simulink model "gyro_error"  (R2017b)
settings: Solver=VariableStepAuto  StartTime=0.0  StopTime=10.0  RelTol=1e-3
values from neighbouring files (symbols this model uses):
  Kg = 15/pi    (= 4.77464829276)    [init.m]
  lg = 0.7    [init.m]
  wg = 200*pi    (= 628.318530718)    [init.m]
undefined symbols (not defined in the file or in its folder): wg2

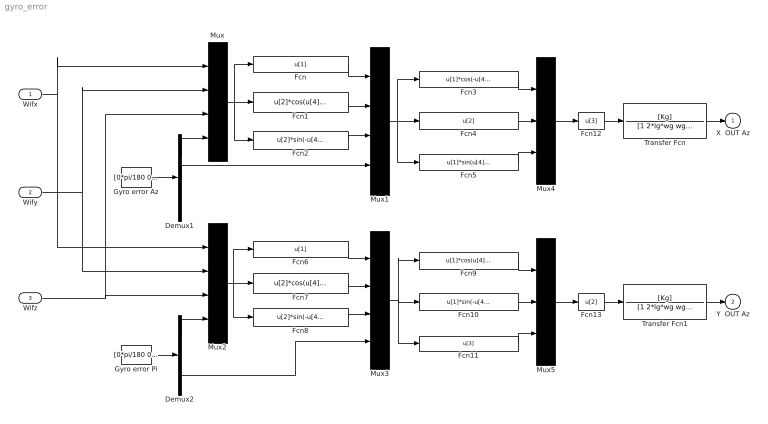
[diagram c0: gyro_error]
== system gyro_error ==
  Wifx : Inport
  Wify : Inport  Port=2
  Wifz : Inport  Port=3
  Demux1 : Demux  Outputs=3
  Demux2 : Demux  Outputs=3
  Fcn : Fcn  Expr=u[1]
  Fcn1 : Fcn  Expr=u[2]*cos(u[4])+u[3]*sin(u[4])
  Fcn10 : Fcn  Expr=u[1]*sin(-u[4])+u[2]*cos(u[4])
  Fcn11 : Fcn  Expr=u[3]
  Fcn12 : Fcn  Expr=u[3]
  Fcn13 : Fcn  Expr=u[2]
  Fcn2 : Fcn  Expr=u[2]*sin(-u[4])+u[3]*cos(u[4])
  Fcn3 : Fcn  Expr=u[1]*cos(-u[4])+u[3]*sin(-u[4])
  Fcn4 : Fcn  Expr=u[2]
  Fcn5 : Fcn  Expr=u[1]*sin(u[4])+u[3]*cos(u[4])
  Fcn6 : Fcn  Expr=u[1]
  Fcn7 : Fcn  Expr=u[2]*cos(u[4])+u[3]*sin(u[4])
  Fcn8 : Fcn  Expr=u[2]*sin(-u[4])+u[3]*cos(u[4])
  Fcn9 : Fcn  Expr=u[1]*cos(u[4])+u[2]*sin(u[4])
  Gyro error Az : Constant  Value=[0*pi/180 0*pi/180 0*pi/180]'
  Gyro error Pi : Constant  Value=[0*pi/180 0*pi/180 0*pi/180]'
  Mux{,1..3} (4 alike) : Mux
  Mux4 : Mux  Inputs=3
  Mux5 : Mux  Inputs=3
  Transfer Fcn : TransferFcn  Numerator=[Kg]  Denominator=[1 2*lg*wg wg2]
  Transfer Fcn1 : TransferFcn  Numerator=[Kg]  Denominator=[1 2*lg*wg wg2]
  X  OUT Az : Outport
  Y  OUT Az : Outport  Port=2
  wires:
  Gyro error Az/1 -> Demux1/1
  Gyro error Pi/1 -> Demux2/1
  Mux/1 -> Fcn/1, Fcn1/1, Fcn2/1
  Wifx/1 -> Mux/1, Mux2/1
  Wify/1 -> Mux/2, Mux2/2
  Wifz/1 -> Mux/3, Mux2/3
  Demux1/1 -> Mux/4
  Mux1/1 -> Fcn3/1, Fcn4/1, Fcn5/1
  Fcn/1 -> Mux1/1
  Fcn1/1 -> Mux1/2
  Fcn2/1 -> Mux1/3
  Demux1/2 -> Mux1/4
  Mux3/1 -> Fcn9/1, Fcn10/1, Fcn11/1
  Demux2/1 -> Mux2/4
  Fcn6/1 -> Mux3/1
  Mux2/1 -> Fcn8/1, Fcn7/1, Fcn6/1
  Fcn7/1 -> Mux3/2
  Fcn8/1 -> Mux3/3
  Demux2/3 -> Mux3/4
  Fcn3/1 -> Mux4/1
  Fcn4/1 -> Mux4/2
  Fcn5/1 -> Mux4/3
  Fcn9/1 -> Mux5/1
  Fcn10/1 -> Mux5/2
  Fcn11/1 -> Mux5/3
  Mux4/1 -> Fcn12/1
  Mux5/1 -> Fcn13/1
  Fcn12/1 -> Transfer Fcn/1
  Fcn13/1 -> Transfer Fcn1/1
  Transfer Fcn/1 -> X  OUT Az/1
  Transfer Fcn1/1 -> Y  OUT Az/1
